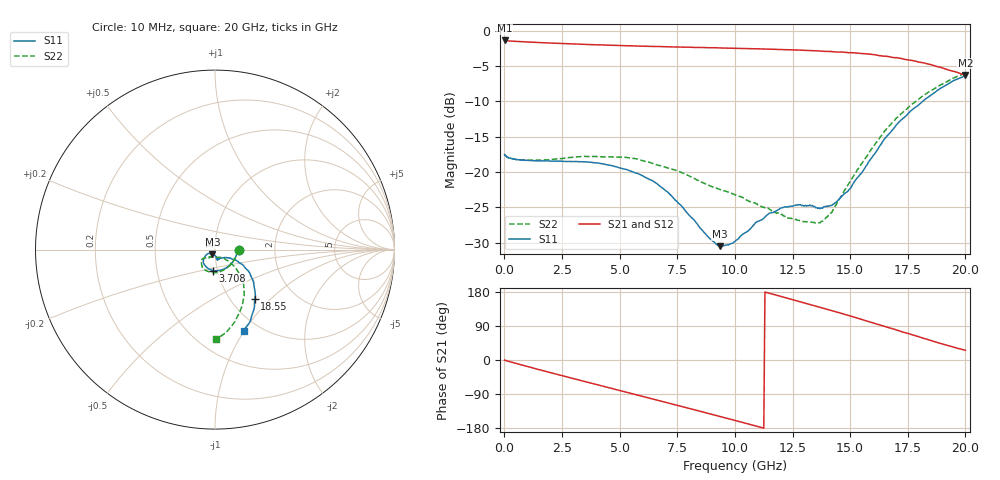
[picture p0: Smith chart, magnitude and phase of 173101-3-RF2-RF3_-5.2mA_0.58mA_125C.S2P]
!  2-Port S-parameters saved by WinCal
! VAR MeasName=S-Parameters (CALIBRATED_DATA) read from VNA (N5242A)
! VAR MeasDate=2017-7-20 10:56:45
! VAR NAME=173101-3-RF2-RF3_-5.2mA_0.58mA_125C
! VAR FILENAME=173101-3-RF2-RF3_-5.2mA_0.58mA_125C.S2P
! VAR DATE=2017-7-20 10:56:45
! VAR PHYS_PORTS=1,2
# Hz S DB R 50
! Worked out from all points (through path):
!   401 points, 10 MHz to 20 GHz, reference 50 ohm
!   highest |S21| = -1.39 dB at 10 MHz (marker M1); lowest = -6.3 dB at 20 GHz (marker M2)
!   group delay of S21, straight-line fit = 46 ps
!   lowest |S11| = -30.5 dB at 9.355 GHz (marker M3), VSWR 1.06, Z = 48.5 - j2.51 ohm
!   |S11| at or under -10 dB: start of sweep to 18.15 GHz
!   |S22| runs from -27.2 to -6.0 dB; largest |S21 - S12| = 0.006
!   S11 on the Smith chart (normalised r, x): 10 MHz: 1.31, -0.01; 3.708 GHz: 0.95, -0.23; 18.55 GHz: 1.29, -0.81; 20 GHz: 0.84, -0.99
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1e7  -17.56 -1.1  -1.39 -0.2  -1.39 -0.2  -17.55 -1.0
1.559225e9  -18.45 -46.2  -1.69 -26.3  -1.69 -26.3  -18.34 -46.6
3.358325e9  -18.57 -88.8  -1.94 -54.8  -1.94 -54.8  -17.81 -86.9
3.70815e9  -18.62 -95.1  -1.97 -60.2  -1.97 -60.3  -17.83 -92.9
5.10745e9  -19.52 -120.9  -2.11 -82.2  -2.12 -82.2  -17.92 -115.3
6.70665e9  -21.90 -140.3  -2.25 -107.1  -2.24 -107.1  -19.07 -132.3
7.956025e9  -25.91 -150.4  -2.34 -126.7  -2.36 -126.7  -20.48 -141.7
8.8056e9  -29.07 -142.8  -2.41 -140.2  -2.42 -140.2  -21.80 -143.5
9.355325e9  -30.51 -119.8  -2.46 -149.1  -2.44 -149.1  -22.49 -141.2
1.0005e10  -29.83 -93.5  -2.51 -159.5  -2.51 -159.5  -23.24 -137.9
1.090455e10  -27.16 -79.0  -2.57 -174.0  -2.58 -174.0  -24.47 -129.9
1.165418e10  -25.76 -79.1  -2.63 173.6  -2.64 173.6  -25.57 -125.4
1.265368e10  -24.67 -78.5  -2.74 156.8  -2.75 156.9  -26.71 -113.3
1.335332e10  -24.74 -73.0  -2.84 145.0  -2.82 145.0  -27.11 -93.6
1.38031e10  -25.15 -64.3  -2.92 137.2  -2.91 137.2  -26.98 -74.5
1.445278e10  -24.06 -47.8  -3.04 126.0  -3.04 126.1  -24.28 -49.5
1.495252e10  -22.51 -36.0  -3.13 117.1  -3.11 116.9  -21.58 -43.2
1.570215e10  -19.12 -28.9  -3.28 103.4  -3.32 103.4  -17.87 -40.7
1.670165e10  -14.54 -29.7  -3.68 84.8  -3.74 84.6  -13.47 -46.5
1.76012e10  -11.44 -38.3  -4.17 68.4  -4.17 68.3  -10.63 -56.3
1.855072e10  -9.03 -51.1  -4.85 50.4  -4.91 50.5  -8.42 -69.2
2e10  -6.36 -70.7  -6.28 25.5  -6.33 26.1  -6.01 -89.3
